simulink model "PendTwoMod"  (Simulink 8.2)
settings: Solver=VariableStepDiscrete  StartTime=0.0  StopTime=simParam_time  MaxStep=Ts  RelTol=1e-3
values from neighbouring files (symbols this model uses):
  simParam_disturbance = 1    [ConfigureSimParams.m]
  Ts = linMod_sim.Ts    [RunSimulation.m]
undefined symbols (not defined in the file or in its folder): A_, B_, C_, deltas_, F_, flag_occReset_, flag_simPacketDrop_, L_, p_pend2M, period_reset_, prob_packetDrop_
libraries: cstblocks x1

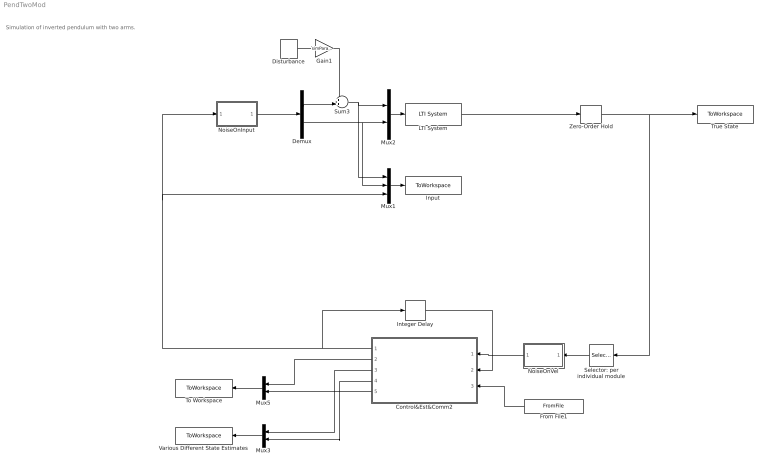
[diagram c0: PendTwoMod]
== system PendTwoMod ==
  note: Simulation of inverted pendulum with two arms.
  Control&Est&Comm2 : MATLAB Function  TreatAsAtomicUnit=on
  Demux : Demux  Outputs=2
  Disturbance : DiscretePulseGenerator  Amplitude=0.5  Period=20000  PulseWidth=10  PhaseDelay=4000  SampleTime=1/100
  From File1 : FromFile  FileName=temp_rand_drop.mat  SampleTime=Ts
  Gain1 : Gain  Gain=simParam_disturbance
  Input : ToWorkspace  VariableName=simout_u  SampleTime=-1  SaveFormat=Timeseries
  Integer Delay : Delay  DelayLength=1  InputProcessing=Inherited  SampleTime=Ts
  LTI System : cstblocks/LTI System  sys=linMod_sim  IC=[p_pend2M.ICAngleUpperMod, 0, p_pend2M.ICAngleLowerMod, 0, p_pend2M.ICAnglePend, 0]
  Mux1 : Mux  Inputs=3
  Mux2 : Mux  Inputs=2
  Mux3 : Mux  Inputs=2
  Mux5 : Mux  Inputs=2
  NoiseOnInput : Subsystem
  NoiseOnVel : Subsystem
  Selector: per individual module : Selector  InputPortWidth=6  IndexOptions=Index vector (dialog)  Indices=[1 3 6]  OutputSizes=1
  Sum3 : Sum  Inputs=++|
  To Workspace : ToWorkspace  VariableName=simout_gamma  SampleTime=-1  SaveFormat=Timeseries
  True State : ToWorkspace  VariableName=simout_x  SampleTime=-1  SaveFormat=Timeseries
  Various Different State Estimates : ToWorkspace  VariableName=simout_xhats  SampleTime=1/100  SaveFormat=Timeseries
  Zero-Order Hold : ZeroOrderHold  SampleTime=Ts
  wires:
  Selector: per individual module/1 -> NoiseOnVel/1(In1)
  Control&Est&Comm2/5(gamma_ex) -> Mux5/2
  Control&Est&Comm2/2(gamma_k) -> Mux5/1
  Demux/1 -> Sum3/2
  Sum3/1 -> Mux1/1, Mux2/1
  Disturbance/1 -> Gain1/1
  Mux3/1 -> Various Different State Estimates/1
  Mux5/1 -> To Workspace/1
  NoiseOnVel/1(Out1) -> Control&Est&Comm2/1(y_k)
  Integer Delay/1 -> Control&Est&Comm2/2(u_km1)
  NoiseOnInput/1(Out1) -> Demux/1
  Control&Est&Comm2/1(u_k) -> Integer Delay/1, Mux1/3, NoiseOnInput/1(In1)
  Mux2/1 -> LTI System/1
  LTI System/1 -> Zero-Order Hold/1
  Mux1/1 -> Input/1
  Demux/2 -> Mux1/2, Mux2/2
  Control&Est&Comm2/3(x_hat1_k) -> Mux3/1
  Control&Est&Comm2/4(x_hat2_k) -> Mux3/2
  Zero-Order Hold/1 -> True State/1, Selector: per individual module/1
  Gain1/1 -> Sum3/1
  From File1/1 -> Control&Est&Comm2/3(rand3)

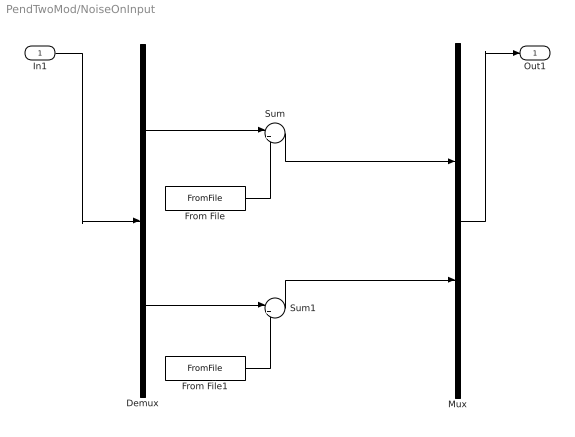
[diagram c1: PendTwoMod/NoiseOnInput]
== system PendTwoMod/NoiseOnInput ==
  In1 : Inport
  Demux : Demux  Outputs=2
  From File : FromFile  FileName=temp_rand_u1.mat  SampleTime=Ts
  From File1 : FromFile  FileName=temp_rand_u2.mat  SampleTime=Ts
  Mux : Mux  Inputs=2
  Sum : Sum  Inputs=|++
  Sum1 : Sum  Inputs=|++
  Out1 : Outport
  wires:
  Mux/1 -> Out1/1
  In1/1 -> Demux/1
  Demux/1 -> Sum/1
  Sum/1 -> Mux/1
  Demux/2 -> Sum1/1
  Sum1/1 -> Mux/2
  From File/1 -> Sum/2
  From File1/1 -> Sum1/2

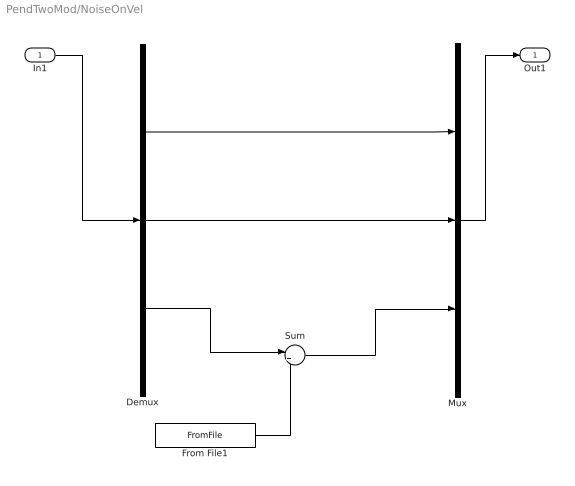
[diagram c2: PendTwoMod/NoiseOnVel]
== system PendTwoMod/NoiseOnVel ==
  In1 : Inport
  Demux : Demux  Outputs=3
  From File1 : FromFile  FileName=temp_rand_gyro.mat  SampleTime=Ts
  Mux : Mux  Inputs=3
  Sum : Sum  Inputs=|++
  Out1 : Outport
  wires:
  Sum/1 -> Mux/3
  In1/1 -> Demux/1
  Mux/1 -> Out1/1
  Demux/3 -> Sum/1
  Demux/1 -> Mux/1
  Demux/2 -> Mux/2
  From File1/1 -> Sum/2

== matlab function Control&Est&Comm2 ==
function [u_k, gamma_k, x_hat1_k, x_hat2_k, gamma_ex]  = fcn(y_k,u_km1, rand3, L_, F_, A_, B_, deltas_, flag_occReset_, period_reset_, flag_simPacketDrop_, prob_packetDrop_, C_)
%#codegen
% Simulation Example.
% Implementation of control, estimation, and communication for both control
% agents.
%
% Input signals:
%   y_k: sensor measurements
%           y_k(1)      angle agent 1 (only known to agent 1)
%           y_k(2)      angle agent 2 (only known to agent 2)
%           y_k(3)      ang vel pendulum (measured/known by agent 2)
%   u_km1: previous commands (known by both)
%   rand3: uniform random number vector with 3 elements, each in [0,1]
%
% Output signals:
%   u_k: control commands
%   gamma_k: sending decisions for y_k(1:3); gamma_k(2)=1 means that y_k(2)
%           was sent
%   xhat_1_k: estimate by agent 1
%   xhat_2_k: estimate by agent 2
%   gamma_ex: extra packets sent to account for synchronous averaging
%
% --
% Supplementary material to:
% Sebastian Trimpe, "Stability Analysis of Distributed Event-Based State
% Estimation", IEEE Conference on Decision and Control (CDC), 2014.
%
% Copyright:
% Sebastian Trimpe
% Max-Planck-Institute for Intelligent Systems
% Autonomous Motion Department
% strimpe(at)tuebingen.mpg.de
%

% Revision history
% [21.03.14]   first version to be published
% [14.09.14]   update (using TSS model), final submission version
%              random numbers as input signal



%% User configuration (from block mask)
% Synchronous averaging
flag_occReset = flag_occReset_;     % enable/disable = true/false
period_reset = period_reset_;       % period K, []=samples

% Simulate packet drops
flag_simPacketDrop = flag_simPacketDrop_;   % enable/disable = true/false
prob_packetDrop = prob_packetDrop_;         % packet drop probability

% System model (for estimation)
A = A_;
n = length(A);
B = B_(:,1:2);
Bprev = B_(:,3:4);
C = C_;
    
% sending thresholds
deltas = deltas_;

% Observer gain
L = L_;

% State-feedback controller gain
F = F_;



%% Variables
% Persistent variables: to be kept in-between calls.
persistent x_hat1;
if isempty(x_hat1)
   x_hat1 = zeros(4,1);
end
persistent x_hat2;
if isempty(x_hat2)
   x_hat2 = zeros(4,1);
end
persistent u_prev;
if isempty(u_prev)
   u_prev = zeros(2,1);
end

persistent counter_k;
if isempty(counter_k)
    %rand('seed',floor(sum(clock)));
    counter_k = 0;
end;

% Extra communication due to synchronous resetting.
gamma_ex = zeros(2,1);      % [Agent 1, Agent 2]

% Disturbance variable
d_k = zeros(8,1);


%% Estimation: prediction step
% Agent 1
x_pred1 = A*x_hat1 + B*u_km1 + Bprev*u_prev;

% Agent 2
x_pred2 = A*x_hat2 + B*u_km1 + Bprev*u_prev;

% Keep input for next step 
u_prev = u_km1;


%% Sending decisions
gamma = zeros(3,1);

% Agent 1 responsibe for y_k(1)
for i=1:1
    gamma(i) = (norm(y_k(i)-C(i,:)*x_pred1) >= deltas(i));
end;

% Agent 2 responsibe for y_k(2:3)
for i=2:3
    gamma(i) = (norm(y_k(i)-C(i,:)*x_pred2) >= deltas(i));
end;



%% Simulate packet drop
if flag_simPacketDrop
    % Agent 1: relevant measurements y(2:3) (received from Agent 2)
    for i=2:3
        if gamma(i)
            if rand3(i)<=prob_packetDrop     % old: myrand<=prob_packetDrop
                % If measurement is sent AND is dropped
                % Add corresponding term to disturbance
                d_k(1:4) = d_k(1:4) -L(:,i)*(y_k(i)-C(i,:)*x_pred1);
% Testing:
%                 disp('1');
%             else
%                 disp('0');
            end;
        end;
    end;
    
    % Agent 2: relevant measurements y(1) (received from Agent 1)
    for i=1:1
        if gamma(i)
            if rand3(i)<=prob_packetDrop    % && rand<=prob_packetDrop  %
                % If measurement is sent AND is dropped
                % Add corresponding term to disturbance
                d_k(5:8) = d_k(5:8) -L(:,i)*(y_k(i)-C(i,:)*x_pred2);
            end;
        end;
    end;
end;


%% Estimation: measurement update
% Module 1
indRcv1 = find(gamma);   % indices of received measurements
x_hat1 = x_pred1 + L(:,indRcv1)*(y_k(indRcv1)-C(indRcv1,:)*x_pred1)+d_k(1:4);

% Module 2
indRcv2 = find(gamma);   % indices of received measurements
x_hat2 = x_pred2 + L(:,indRcv2)*(y_k(indRcv2)-C(indRcv2,:)*x_pred2)+d_k(5:8);


%% Synchronous averaging: Occationally reset x_hat1 with x_hat2
if flag_occReset
    if counter_k==period_reset
        % Reset both with average
        x_hatAvg = (x_hat1+x_hat2)/2;
        x_hat1 = x_hatAvg;
        x_hat2 = x_hatAvg;
        
        % set communication variables accordingly
        % Required communication: each module needs to communicate n
        % numbers.
        gamma_ex = [n n]';
        
        % inc counter
        counter_k = 0;
    end;
    counter_k = counter_k+1;
end;


% full vectors, also including arm velocities (previous input)
x_hat1_k = [x_hat1(1);u_km1(1);x_hat1(2);u_km1(2);x_hat1(3:4)];
x_hat2_k = [x_hat2(1);u_km1(1);x_hat2(2);u_km1(2);x_hat2(3:4)];


%% Control
u1 = F(1,:)*x_hat1_k;
u2 = F(2,:)*x_hat2_k;


%% Output
gamma_k = gamma;
u_k = [u1; u2];
